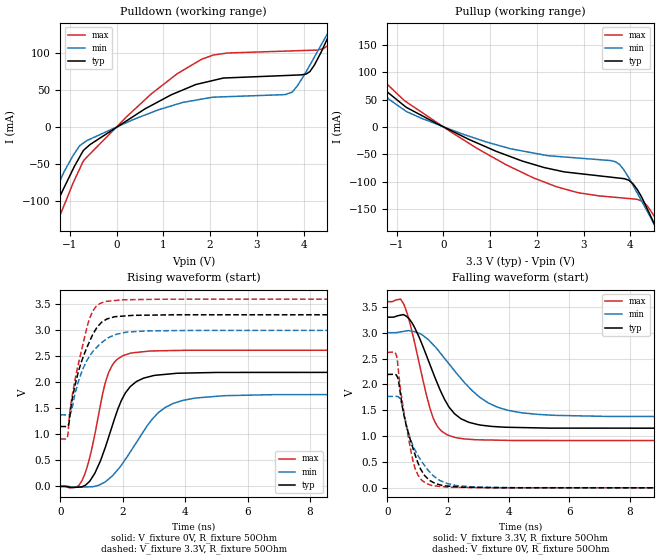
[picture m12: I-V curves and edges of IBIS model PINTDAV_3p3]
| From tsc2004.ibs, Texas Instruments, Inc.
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| Model 3.3 V PINTDAV
[Model]   PINTDAV_3p3
Model_type  Output
Polarity   Non-Inverting
Enable   Active-Low
Vmeas = 1.65
Vref = 1.65
Cref = 15pF
Rref = 50
|   typ   min   max
|   (nom PVT)   (Fast PVT)   (slow PVT)
|   Output High
C_comp   8.01827E-12   8.01827E-12   8.28093E-12
|   Output Low
|C_comp   8.51294E-12   8.63136E-12   8.67118E-12
| Where   nom PVT is  Nominal Process, 3.3V, 25C
|   Fast PVT is Strong Process, 3.6V, -40C
|   Slow PVT is Weak Process, 3.0V, 85C
|C_comp - from L-C Tank method, L = 1nH, peak frequency
|C_comp from frequency method, F = 10 MHz
[Voltage Range]   3.3   3   3.6
[Temperature Range]   30   88   -40
|Ambient Temperature Range 27   85   -40
[Pullup Reference]   3.3   3   3.6
[Pulldown Reference]   0   0   0
[Power Clamp Reference]   3.3   3   3.6
[GND Clamp Reference]   0   0   0
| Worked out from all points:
|   slope of the pulldown table from 0 to 0.495 V, typ, clamps not added: 24.3 ohm
|   slope of the pullup table from 0 to 0.495 V, typ, clamps not added: 23.8 ohm
|   falling waveform, V_fixture 3.3V, R_fixture 50Ohm: 20-80 % time 935ps typ, 1.52ns min, 658ps max; typ from 3.3 V to 1.15 V
|   rising waveform, V_fixture 0V, R_fixture 50Ohm: 20-80 % time 799ps typ, 1.25ns min, 567ps max; typ from 0 V to 2.19 V
|   rising waveform, V_fixture 3.3V, R_fixture 50Ohm: 20-80 % time 648ps typ, 728ps min, 548ps max; typ from 1.15 V to 3.3 V
|   falling waveform, V_fixture 0V, R_fixture 50Ohm: 20-80 % time 595ps typ, 774ps min, 449ps max; typ from 2.19 V to 0 V
[Pulldown]
|   Voltage   I(typ)   I(min)   I(max)
-3.3V     -485.3mA   -406.9mA   -623.5mA
-1.77V    -189.1mA   -157.7mA   -230.4mA
-1.495V   -137.7mA   -113.9mA   -167.5mA
-1.301V   -107.1mA   -85.91mA   -134.2mA
-691.4mV  -30.81mA   -21.06mA   -44.55mA
747.6mV   29.19mA    19.54mA    45mA
1.834V    59.51mA    37.83mA    91.98mA
3.755V    70.01mA    47.05mA    103mA
4.142V    75.5mA     84.45mA    103.8mA
4.624V    135mA      138.9mA    121mA
4.749V    152mA      153.4mA    140.1mA
6.59V     421.2mA    376.9mA    479.5mA
[Pullup]
|   Voltage   I(typ)   I(min)   I(max)
-3.3V     340.9mA    290.7mA    413.8mA
-2.057V   166.4mA    145.5mA    194.4mA
-1.494V   91.32mA    82.68mA    103.5mA
-796.3mV  36.05mA    28.49mA    45.98mA
923.7mV   -36.97mA   -27.67mA   -49.11mA
1.93V     -68.62mA   -47.81mA   -93.37mA
3.688V    -92.96mA   -63.93mA   -128.9mA
4.063V    -104.8mA   -107.7mA   -131.8mA
4.272V    -133.9mA   -140.5mA   -136.9mA
4.577V    -189.1mA   -189.6mA   -173.2mA
4.699V    -212.9mA   -209.7mA   -195.5mA
6.59V     -587.8mA   -525.7mA   -681.8mA
[Ramp]
R_load = 50
|   typ   min   max
dV/dt_r   1.31585/7.94203e-010   1.06072/1.24893e-009   1.57108/5.62891e-010
dV/dt_f   1.28911/9.33525e-010  0.974899/1.512e-009   1.61224/6.53824e-010
[Falling Waveform]
V_fixture = 3.3V
V_fixture_min = 3V
V_fixture_max = 3.6V
R_fixture = 50Ohm
C_fixture = 0F
|   Time   V(typ)   V(min)   V(max)
0s        3.3V       3V         3.6V
526.6ps   3.35V      3.024V     3.568V
882.3ps   3.12V      3.021V     2.852V
1.291ns   2.557V     2.893V     1.791V
1.505ns   2.23V      2.771V     1.361V
1.786ns   1.833V     2.578V     1.098V
2.229ns   1.427V     2.254V     974.6mV
3.334ns   1.195V     1.64V      925.4mV
4.958ns   1.159V     1.421V     915.2mV
20ns      1.151V     1.375V     912.9mV
[Rising Waveform]
V_fixture = 0V
V_fixture_min = 0V
V_fixture_max = 0V
R_fixture = 50Ohm
C_fixture = 0F
|   Time   V(typ)   V(min)   V(max)
0s        48.42nV    64.81nV    32.67nV
591.8ps   -13.25mV   -15.3mV    21.13mV
947.2ps   106.7mV    -7.891mV   577.6mV
1.365ns   627.7mV    63.98mV    1.813V
1.542ns   941.8mV    139.1mV    2.183V
1.952ns   1.649V     406.4mV    2.494V
2.249ns   1.924V     670.6mV    2.561V
3.156ns   2.142V     1.426V     2.607V
4.351ns   2.182V     1.7V       2.617V
20ns      2.193V     1.768V     2.618V
[Rising Waveform]
V_fixture = 3.3V
V_fixture_min = 3V
V_fixture_max = 3.6V
R_fixture = 50Ohm
C_fixture = 0F
|   Time   V(typ)   V(min)   V(max)
0s        1.151V     1.375V     912.9mV
228.1ps   1.159V     1.375V     955.4mV
302.6ps   1.349V     1.387V     1.441V
446.5ps   1.886V     1.724V     1.983V
651.1ps   2.358V     2.151V     2.551V
920.9ps   2.768V     2.494V     3.206V
1.129ns   3.016V     2.652V     3.45V
1.445ns   3.202V     2.82V      3.556V
2.792ns   3.292V     2.99V      3.595V
20ns      3.3V       3V         3.6V
[Falling Waveform]
|Gnd
V_fixture = 0V
V_fixture_min = 0V
V_fixture_max = 0V
R_fixture = 50Ohm
C_fixture = 0F
|   Time   V(typ)   V(min)   V(max)
0s        2.193V     1.768V     2.618V
308.5ps   2.171V     1.769V     2.542V
421.7ps   1.857V     1.718V     1.957V
535.3ps   1.444V     1.457V     1.51V
911.9ps   645.9mV    732.8mV    382.2mV
1.231ns   237.2mV    429.1mV    106.1mV
1.484ns   114.6mV    251.5mV    42.84mV
1.971ns   35.6mV     83.74mV    14.39mV
2.974ns   8.467mV    12.96mV    4.538mV
20ns      22.8nV     16.66nV    15.94nV
